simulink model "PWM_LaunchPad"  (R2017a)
settings: Solver=FixedStepDiscrete  StartTime=0.0  StopTime=inf  RelTol=1e-3  EnableMultiTasking=on
undefined symbols (not defined in the file): A, Compare, conversion, DCAEVT1, DCAEVT1FILT, Digital, Event, Filtered, GPTRIP1SEL, GPTRIP2SEL, input, Module, of, start, Trip, TZ1, TZ2, version, Zone
libraries: c2802xlib x5, idelinklib_common x1

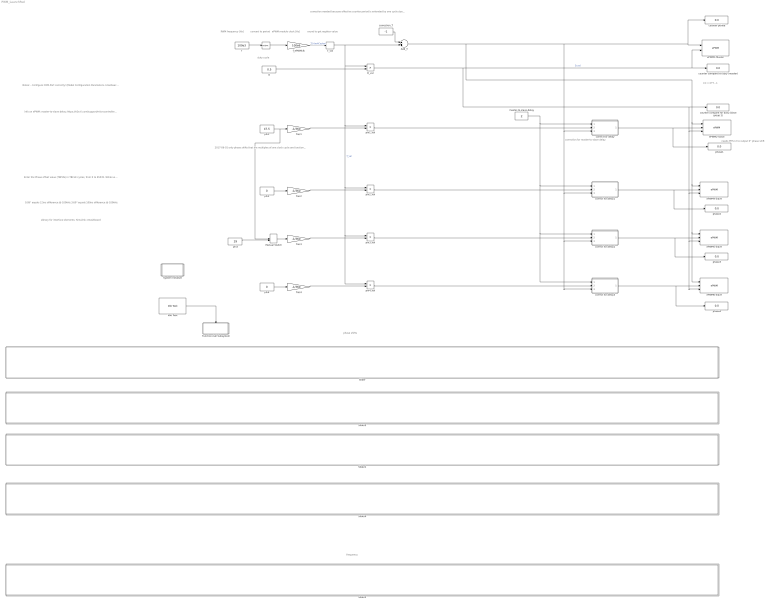
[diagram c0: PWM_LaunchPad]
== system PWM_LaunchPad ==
  note: 2017-06-01 only phase shifts that are multiples of one clock cycle are functioning correctly
  note: correction for master-to-slave delay
  note: needs PHS=2 to output 0° phase shift
  note: info on ePWM: master-to-slave delay: https://e2e.ti.com/support/microcontrollers/c2000/f/171/p/279536/976108 lagging phase-shift: http://e2e.ti.com/support/microcontrollers/c2000/f/171/p/582633/2143131
  note: PWM frequency [Hz]
  note: convert to period
  note: CC = D*T - 1
  note: phase shifts
  note: Library for interface elements: Simulink->Dashboard
  note: Notes: - Configure COM-Port correctly! (Model Configuration Parameters->Hardware Implementation->Groups:External Mode->Serial port) COM-Port Number taken from Windows device manager - In model settings -> Hardware Implementation, disable "Boot from flash" (unnecessary, only slows down program download)
  note: 0.09° equals 2.5ns difference @ 100kHz 3.60° equals 100ns difference @ 100kHz
  note: Enter the Phase offset value (TBPHS) in TBCLK cycles, from 0 to 65535. While using HRPWM, you may enter decimal values The Extension Register for the HRPWM Period (TBPRDHR) provides an 8 bit representation of the decimal part
  note: frequency
  note: correction needed because effective counter period is extended by one cycle due to counter reload See ePWM RefGuide, p. 89, Example 14
  note: ePWM module clock [Hz]
  note: round to get register value
  note: duty cycle
  Add_T : Sum
  D : Constant  Value=0.5
  D_val : Product
  Function-Call Subsystem : Subsystem  TreatAsAtomicUnit=on
  Idle Task : idelinklib_common/Idle Task  tasknumbers=[1]  taskpriorities=100017  taskpreempts=[0]  showinput=off  simPriority=0
  Manual Switch : ManualSwitch
  Slider : Subsystem  DialogController=hmiCreateDDGDialog  IsWebBlock=on
  Slider1 : Subsystem  DialogController=hmiCreateDDGDialog  IsWebBlock=on
  Slider2 : Subsystem  DialogController=hmiCreateDDGDialog  IsWebBlock=on
  Slider3 : Subsystem  DialogController=hmiCreateDDGDialog  IsWebBlock=on
  Slider4 : Subsystem  DialogController=hmiCreateDDGDialog  IsWebBlock=on
  System Initialize : Subsystem
  T : Math  Operator=reciprocal
  T_val : Rounding
  correct for delay : Subsystem
  correct for delay1 : Subsystem
  correct for delay2 : Subsystem
  correct for delay3 : Subsystem
  correction_T : Constant  Value=-1
  counter compare for duty (master) : Display
  counter compare for duty (slave group 1) : Display
  counter period : Display
  ePWM1-Master : c2802xlib/ePWM  useModule=ePWM1  ePWMxLINKTBPRD=Not Linked  periodUnits=Clock cycles  timerSource=Input port  timerPeriod_clk=0  timerPeriod_sec=10e-3  tbshadow=Counter equals to zero  countingMode=Up  phaseActiveEnable=Disable  phaseDirection=Count down after sync  phaseActive=0  synchronizationEnable=off  dcaevt1Sync=off  dcbevt1Sync=off  synchronizationOption=Counter equals to zero (CTR=Zero)  clockPrescale=1  HSclockPrescale=1  enswap=off  ePWMxAStatus=on  ePWMxAactionLogic1=Set  ePWMxAactionLogic2=Do nothing  ePWMxAactionLogic3=Clear  ePWMxAactionLogic4=Clear  ePWMxAactionLogic5=Do nothing  ePWMxAactionLogic6=Do nothing  ePWMxALoadMode=Load on counter equals to zero (CTR=Zero)  ePWMxACSFenable=off  ePWMxACSFvalue=Forcing disable  ePWMxASFreload=Zero  ePWMxBStatus=off  ePWMxBactionLogic1=Do nothing  ePWMxBactionLogic2=Do nothing  ePWMxBactionLogic3=Do nothing  ePWMxBactionLogic4=Do nothing  ePWMxBactionLogic5=Do nothing  ePWMxBactionLogic6=Do nothing  ePWMxBLoadMode=Load on counter equals to zero (CTR=Zero)  ePWMxBCSFenable=off  ePWMxBCSFvalue=Forcing disable  ePWMxBSFreload=Zero  ePWNxBOutWay=off  ePWMxLINKCMPA=Not Linked  CMPAUnits=Clock cycles  CMPASource=Input port  CMPAValue_per=50  CMPAValue_clk=0  enCMPAshadow=Counter equals to zero  ePWMxLINKCMPB=Not Linked  CMPBUnits=Clock cycles  CMPBSource=Specify via dialog  CMPBValue_per=50  CMPBValue_clk=0  enCMPBshadow=Counter equals to zero  ePWMxLINKCMPC=Not Linked  CMPCUnits=Clock cycles  CMPCSource=Specify via dialog  CMPCValue_per=50  CMPCValue_clk=0  enCMPCshadow=Counter equals to zero  ePWMxLINKCMPD=Not Linked  CMPDUnits=Clock cycles  CMPDSource=Specify via dialog  CMPDValue_per=50  CMPDValue_clk=0  enCMPDshadow=Counter equals to zero  enableDBePWMxA=off  enableDBePWMxB=off  enhalfcycle=off  DBpolarity=Active high (AH)  DBedgeDelay=Positive  DBSource_ePWMxA=ePWMxA  DBSource_ePWMxB=ePWMxA  DBperiodSource=Specify via dialog  REDperiod=0  FEDperiod=0  adcstartModuleA=off  adcrequestEventA=First event  adcstartEventA=Digital Compare Module A Event 1 start of conversion (DCAEVT1.soc)  adcstartEventA_type2=Counter equals to period (CTR=PRD)  adcstartModuleB=off  adcrequestEventB=First event  adcstartEventB=Counter equals to zero (CTR=Zero)  adcstartEventB_type2=Counter equals to zero (CTR=Zero)  intEn=off  intPrd=First event  intSel=Counter equals to zero (CTR=Zero)  intSel_type2=Counter equals to zero (CTR=Zero)  hrpe=off  enHRPWM=on  HRPWM_LoadMode=Counter equals to zero (CTR=ZERO)  HRPWM_CTLMode=Phase control mode  HRPWM_EDGMode=Both edge  hrpeb=off  enHRPWMB=off  HRPWM_LoadModeB=Counter equals to zero (CTR=ZERO)  HRPWM_CTLModeB=Duty or Period control mode  HRPWM_EDGModeB=Both edge  enSFO=on  enautoconv=on  chopperEnable=off  chopperFrequency=1  chopperFirstwidth=1  chopperDuty=12.5%  tripZonesource=Specify via dialog  tzselOSHT1=off  tzselOSHT2=off  tzselOSHT3=off  tzselOSHDCAEV1=off  tzselOSHDCBEV1=off  tzselCBC1=off  tzselCBC2=off  tzselCBC3=off  tzselCBCDCAEV2=off  tzselCBCDCBEV2=off  tzselOSHT4=off  tzselOSHT5=off  tzselOSHT6=off  tzselCBC4=off  tzselCBC5=off  tzselCBC6=off  enTzOstIntr=off  enTzCbcIntr=off  enTzDCAEVT1Intr=off  enTzDCAEVT2Intr=off  enTzDCBEVT1Intr=off  enTzDCBEVT2Intr=off  ePWMxAforced=No action  ePWMxBforced=No action  DCAEVT1forced=No action  DCBEVT1forced=No action  DCAEVT2forced=No action  DCBEVT2forced=No action  dcah=Trip Zone 1 input (TZ1)  dcal=Trip Zone 2 input (TZ2)  dcbh=Trip Zone 1 input (TZ1)  dcbl=Trip Zone 2 input (TZ2)  dcah_type2=GPTRIP1SEL/(TZ1)  dcal_type2=GPTRIP2SEL/(TZ2)  dcbh_type2=GPTRIP1SEL/(TZ1)  dcbl_type2=GPTRIP2SEL/(TZ2)  gendcaevt1=Event disabled  gendcaevt2=Event disabled  gendcbevt1=Event disabled  gendcbevt2=Event disabled  dcaevt1src=DCAEVT1 with sync  dcaevt2src=DCAEVT2 with sync  dcbevt1src=DCBEVT1 with sync  dcbevt2src=DCBEVT2 with sync  pulsesel=Counter equals to zero (CTR=Zero)  blankinv=off  blankoffset=0  blankwidth=0  evsrcsel=Filtered version of DCAEVT1 (DCAEVT1FILT)  encape=off  PwmType=C2000_Type4
  ePWM2-Slave : c2802xlib/ePWM  useModule=ePWM2  ePWMxLINKTBPRD=Not Linked  periodUnits=Clock cycles  timerSource=Input port  timerPeriod_clk=500  timerPeriod_sec=10e-3  tbshadow=Counter equals to zero  countingMode=Up  phaseActiveEnable=Set counter to phase value specified via input port  phaseDirection=Count down after sync  phaseActive=0  synchronizationEnable=off  dcaevt1Sync=off  dcbevt1Sync=off  synchronizationOption=Pass through (EPWMxSYNCI or SWFSYNC)  clockPrescale=1  HSclockPrescale=1  enswap=off  ePWMxAStatus=on  ePWMxAactionLogic1=Set  ePWMxAactionLogic2=Do nothing  ePWMxAactionLogic3=Clear  ePWMxAactionLogic4=Clear  ePWMxAactionLogic5=Do nothing  ePWMxAactionLogic6=Do nothing  ePWMxALoadMode=Load on counter equals to zero (CTR=Zero)  ePWMxACSFenable=off  ePWMxACSFvalue=Forcing disable  ePWMxASFreload=Zero  ePWMxBStatus=off  ePWMxBactionLogic1=Do nothing  ePWMxBactionLogic2=Do nothing  ePWMxBactionLogic3=Do nothing  ePWMxBactionLogic4=Do nothing  ePWMxBactionLogic5=Do nothing  ePWMxBactionLogic6=Do nothing  ePWMxBLoadMode=Load on counter equals to zero (CTR=Zero)  ePWMxBCSFenable=off  ePWMxBCSFvalue=Forcing disable  ePWMxBSFreload=Zero  ePWNxBOutWay=off  ePWMxLINKCMPA=Not Linked  CMPAUnits=Clock cycles  CMPASource=Input port  CMPAValue_per=50  CMPAValue_clk=500  enCMPAshadow=Counter equals to zero  ePWMxLINKCMPB=Not Linked  CMPBUnits=Clock cycles  CMPBSource=Specify via dialog  CMPBValue_per=50  CMPBValue_clk=0  enCMPBshadow=Counter equals to zero  ePWMxLINKCMPC=Not Linked  CMPCUnits=Clock cycles  CMPCSource=Specify via dialog  CMPCValue_per=50  CMPCValue_clk=0  enCMPCshadow=Counter equals to zero  ePWMxLINKCMPD=Not Linked  CMPDUnits=Clock cycles  CMPDSource=Specify via dialog  CMPDValue_per=50  CMPDValue_clk=0  enCMPDshadow=Counter equals to zero  enableDBePWMxA=off  enableDBePWMxB=off  enhalfcycle=off  DBpolarity=Active high (AH)  DBedgeDelay=Positive  DBSource_ePWMxA=ePWMxA  DBSource_ePWMxB=ePWMxA  DBperiodSource=Specify via dialog  REDperiod=0  FEDperiod=0  adcstartModuleA=off  adcrequestEventA=First event  adcstartEventA=Digital Compare Module A Event 1 start of conversion (DCAEVT1.soc)  adcstartEventA_type2=Counter equals to period (CTR=PRD)  adcstartModuleB=off  adcrequestEventB=First event  adcstartEventB=Counter equals to zero (CTR=Zero)  adcstartEventB_type2=Counter equals to zero (CTR=Zero)  intEn=off  intPrd=First event  intSel=Counter equals to zero (CTR=Zero)  intSel_type2=Counter equals to zero (CTR=Zero)  hrpe=off  enHRPWM=on  HRPWM_LoadMode=Counter equals to zero (CTR=ZERO)  HRPWM_CTLMode=Phase control mode  HRPWM_EDGMode=Both edge  hrpeb=off  enHRPWMB=off  HRPWM_LoadModeB=Counter equals to zero (CTR=ZERO)  HRPWM_CTLModeB=Duty or Period control mode  HRPWM_EDGModeB=Both edge  enSFO=on  enautoconv=on  chopperEnable=off  chopperFrequency=1  chopperFirstwidth=1  chopperDuty=12.5%  tripZonesource=Specify via dialog  tzselOSHT1=off  tzselOSHT2=off  tzselOSHT3=off  tzselOSHDCAEV1=off  tzselOSHDCBEV1=off  tzselCBC1=off  tzselCBC2=off  tzselCBC3=off  tzselCBCDCAEV2=off  tzselCBCDCBEV2=off  tzselOSHT4=off  tzselOSHT5=off  tzselOSHT6=off  tzselCBC4=off  tzselCBC5=off  tzselCBC6=off  enTzOstIntr=off  enTzCbcIntr=off  enTzDCAEVT1Intr=off  enTzDCAEVT2Intr=off  enTzDCBEVT1Intr=off  enTzDCBEVT2Intr=off  ePWMxAforced=No action  ePWMxBforced=No action  DCAEVT1forced=No action  DCBEVT1forced=No action  DCAEVT2forced=No action  DCBEVT2forced=No action  dcah=Trip Zone 1 input (TZ1)  dcal=Trip Zone 2 input (TZ2)  dcbh=Trip Zone 1 input (TZ1)  dcbl=Trip Zone 2 input (TZ2)  dcah_type2=GPTRIP1SEL/(TZ1)  dcal_type2=GPTRIP2SEL/(TZ2)  dcbh_type2=GPTRIP1SEL/(TZ1)  dcbl_type2=GPTRIP2SEL/(TZ2)  gendcaevt1=Event disabled  gendcaevt2=Event disabled  gendcbevt1=Event disabled  gendcbevt2=Event disabled  dcaevt1src=DCAEVT1 with sync  dcaevt2src=DCAEVT2 with sync  dcbevt1src=DCBEVT1 with sync  dcbevt2src=DCBEVT2 with sync  pulsesel=Counter equals to zero (CTR=Zero)  blankinv=off  blankoffset=0  blankwidth=0  evsrcsel=Filtered version of DCAEVT1 (DCAEVT1FILT)  encape=off  PwmType=C2000_Type4
  ePWM4-Slave : c2802xlib/ePWM  useModule=ePWM4  ePWMxLINKTBPRD=Not Linked  periodUnits=Clock cycles  timerSource=Input port  timerPeriod_clk=500  timerPeriod_sec=10e-3  tbshadow=Counter equals to zero  countingMode=Up  phaseActiveEnable=Set counter to phase value specified via input port  phaseDirection=Count down after sync  phaseActive=0  synchronizationEnable=off  dcaevt1Sync=off  dcbevt1Sync=off  synchronizationOption=Pass through (EPWMxSYNCI or SWFSYNC)  clockPrescale=1  HSclockPrescale=1  enswap=off  ePWMxAStatus=on  ePWMxAactionLogic1=Set  ePWMxAactionLogic2=Do nothing  ePWMxAactionLogic3=Clear  ePWMxAactionLogic4=Clear  ePWMxAactionLogic5=Do nothing  ePWMxAactionLogic6=Do nothing  ePWMxALoadMode=Load on counter equals to zero (CTR=Zero)  ePWMxACSFenable=off  ePWMxACSFvalue=Forcing disable  ePWMxASFreload=Zero  ePWMxBStatus=off  ePWMxBactionLogic1=Do nothing  ePWMxBactionLogic2=Do nothing  ePWMxBactionLogic3=Do nothing  ePWMxBactionLogic4=Do nothing  ePWMxBactionLogic5=Do nothing  ePWMxBactionLogic6=Do nothing  ePWMxBLoadMode=Load on counter equals to zero (CTR=Zero)  ePWMxBCSFenable=off  ePWMxBCSFvalue=Forcing disable  ePWMxBSFreload=Zero  ePWNxBOutWay=off  ePWMxLINKCMPA=Not Linked  CMPAUnits=Clock cycles  CMPASource=Input port  CMPAValue_per=50  CMPAValue_clk=500  enCMPAshadow=Counter equals to zero  ePWMxLINKCMPB=Not Linked  CMPBUnits=Clock cycles  CMPBSource=Specify via dialog  CMPBValue_per=50  CMPBValue_clk=0  enCMPBshadow=Counter equals to zero  ePWMxLINKCMPC=Not Linked  CMPCUnits=Clock cycles  CMPCSource=Specify via dialog  CMPCValue_per=50  CMPCValue_clk=0  enCMPCshadow=Counter equals to zero  ePWMxLINKCMPD=Not Linked  CMPDUnits=Clock cycles  CMPDSource=Specify via dialog  CMPDValue_per=50  CMPDValue_clk=0  enCMPDshadow=Counter equals to zero  enableDBePWMxA=off  enableDBePWMxB=off  enhalfcycle=off  DBpolarity=Active high (AH)  DBedgeDelay=Positive  DBSource_ePWMxA=ePWMxA  DBSource_ePWMxB=ePWMxA  DBperiodSource=Specify via dialog  REDperiod=0  FEDperiod=0  adcstartModuleA=off  adcrequestEventA=First event  adcstartEventA=Digital Compare Module A Event 1 start of conversion (DCAEVT1.soc)  adcstartEventA_type2=Counter equals to period (CTR=PRD)  adcstartModuleB=off  adcrequestEventB=First event  adcstartEventB=Counter equals to zero (CTR=Zero)  adcstartEventB_type2=Counter equals to zero (CTR=Zero)  intEn=off  intPrd=First event  intSel=Counter equals to zero (CTR=Zero)  intSel_type2=Counter equals to zero (CTR=Zero)  hrpe=off  enHRPWM=on  HRPWM_LoadMode=Counter equals to zero (CTR=ZERO)  HRPWM_CTLMode=Phase control mode  HRPWM_EDGMode=Both edge  hrpeb=off  enHRPWMB=off  HRPWM_LoadModeB=Counter equals to zero (CTR=ZERO)  HRPWM_CTLModeB=Duty or Period control mode  HRPWM_EDGModeB=Both edge  enSFO=on  enautoconv=on  chopperEnable=off  chopperFrequency=1  chopperFirstwidth=1  chopperDuty=12.5%  tripZonesource=Specify via dialog  tzselOSHT1=off  tzselOSHT2=off  tzselOSHT3=off  tzselOSHDCAEV1=off  tzselOSHDCBEV1=off  tzselCBC1=off  tzselCBC2=off  tzselCBC3=off  tzselCBCDCAEV2=off  tzselCBCDCBEV2=off  tzselOSHT4=off  tzselOSHT5=off  tzselOSHT6=off  tzselCBC4=off  tzselCBC5=off  tzselCBC6=off  enTzOstIntr=off  enTzCbcIntr=off  enTzDCAEVT1Intr=off  enTzDCAEVT2Intr=off  enTzDCBEVT1Intr=off  enTzDCBEVT2Intr=off  ePWMxAforced=No action  ePWMxBforced=No action  DCAEVT1forced=No action  DCBEVT1forced=No action  DCAEVT2forced=No action  DCBEVT2forced=No action  dcah=Trip Zone 1 input (TZ1)  dcal=Trip Zone 2 input (TZ2)  dcbh=Trip Zone 1 input (TZ1)  dcbl=Trip Zone 2 input (TZ2)  dcah_type2=GPTRIP1SEL/(TZ1)  dcal_type2=GPTRIP2SEL/(TZ2)  dcbh_type2=GPTRIP1SEL/(TZ1)  dcbl_type2=GPTRIP2SEL/(TZ2)  gendcaevt1=Event disabled  gendcaevt2=Event disabled  gendcbevt1=Event disabled  gendcbevt2=Event disabled  dcaevt1src=DCAEVT1 with sync  dcaevt2src=DCAEVT2 with sync  dcbevt1src=DCBEVT1 with sync  dcbevt2src=DCBEVT2 with sync  pulsesel=Counter equals to zero (CTR=Zero)  blankinv=off  blankoffset=0  blankwidth=0  evsrcsel=Filtered version of DCAEVT1 (DCAEVT1FILT)  encape=off  PwmType=C2000_Type4
  ePWM5-Slave : c2802xlib/ePWM  useModule=ePWM5  ePWMxLINKTBPRD=Not Linked  periodUnits=Clock cycles  timerSource=Input port  timerPeriod_clk=500  timerPeriod_sec=10e-3  tbshadow=Counter equals to zero  countingMode=Up  phaseActiveEnable=Set counter to phase value specified via input port  phaseDirection=Count down after sync  phaseActive=10.25  synchronizationEnable=off  dcaevt1Sync=off  dcbevt1Sync=off  synchronizationOption=Pass through (EPWMxSYNCI or SWFSYNC)  clockPrescale=1  HSclockPrescale=1  enswap=off  ePWMxAStatus=on  ePWMxAactionLogic1=Set  ePWMxAactionLogic2=Do nothing  ePWMxAactionLogic3=Clear  ePWMxAactionLogic4=Clear  ePWMxAactionLogic5=Do nothing  ePWMxAactionLogic6=Do nothing  ePWMxALoadMode=Load on counter equals to zero (CTR=Zero)  ePWMxACSFenable=off  ePWMxACSFvalue=Forcing disable  ePWMxASFreload=Zero  ePWMxBStatus=off  ePWMxBactionLogic1=Do nothing  ePWMxBactionLogic2=Do nothing  ePWMxBactionLogic3=Do nothing  ePWMxBactionLogic4=Do nothing  ePWMxBactionLogic5=Do nothing  ePWMxBactionLogic6=Do nothing  ePWMxBLoadMode=Load on counter equals to zero (CTR=Zero)  ePWMxBCSFenable=off  ePWMxBCSFvalue=Forcing disable  ePWMxBSFreload=Zero  ePWNxBOutWay=off  ePWMxLINKCMPA=Not Linked  CMPAUnits=Clock cycles  CMPASource=Input port  CMPAValue_per=50  CMPAValue_clk=500  enCMPAshadow=Counter equals to zero  ePWMxLINKCMPB=Not Linked  CMPBUnits=Clock cycles  CMPBSource=Specify via dialog  CMPBValue_per=50  CMPBValue_clk=0  enCMPBshadow=Counter equals to zero  ePWMxLINKCMPC=Not Linked  CMPCUnits=Clock cycles  CMPCSource=Specify via dialog  CMPCValue_per=50  CMPCValue_clk=0  enCMPCshadow=Counter equals to zero  ePWMxLINKCMPD=Not Linked  CMPDUnits=Clock cycles  CMPDSource=Specify via dialog  CMPDValue_per=50  CMPDValue_clk=0  enCMPDshadow=Counter equals to zero  enableDBePWMxA=off  enableDBePWMxB=off  enhalfcycle=off  DBpolarity=Active high (AH)  DBedgeDelay=Positive  DBSource_ePWMxA=ePWMxA  DBSource_ePWMxB=ePWMxA  DBperiodSource=Specify via dialog  REDperiod=0  FEDperiod=0  adcstartModuleA=off  adcrequestEventA=First event  adcstartEventA=Digital Compare Module A Event 1 start of conversion (DCAEVT1.soc)  adcstartEventA_type2=Counter equals to period (CTR=PRD)  adcstartModuleB=off  adcrequestEventB=First event  adcstartEventB=Counter equals to zero (CTR=Zero)  adcstartEventB_type2=Counter equals to zero (CTR=Zero)  intEn=off  intPrd=First event  intSel=Counter equals to zero (CTR=Zero)  intSel_type2=Counter equals to zero (CTR=Zero)  hrpe=off  enHRPWM=on  HRPWM_LoadMode=Counter equals to zero (CTR=ZERO)  HRPWM_CTLMode=Phase control mode  HRPWM_EDGMode=Both edge  hrpeb=off  enHRPWMB=off  HRPWM_LoadModeB=Counter equals to zero (CTR=ZERO)  HRPWM_CTLModeB=Duty or Period control mode  HRPWM_EDGModeB=Both edge  enSFO=on  enautoconv=on  chopperEnable=off  chopperFrequency=1  chopperFirstwidth=1  chopperDuty=12.5%  tripZonesource=Specify via dialog  tzselOSHT1=off  tzselOSHT2=off  tzselOSHT3=off  tzselOSHDCAEV1=off  tzselOSHDCBEV1=off  tzselCBC1=off  tzselCBC2=off  tzselCBC3=off  tzselCBCDCAEV2=off  tzselCBCDCBEV2=off  tzselOSHT4=off  tzselOSHT5=off  tzselOSHT6=off  tzselCBC4=off  tzselCBC5=off  tzselCBC6=off  enTzOstIntr=off  enTzCbcIntr=off  enTzDCAEVT1Intr=off  enTzDCAEVT2Intr=off  enTzDCBEVT1Intr=off  enTzDCBEVT2Intr=off  ePWMxAforced=No action  ePWMxBforced=No action  DCAEVT1forced=No action  DCBEVT1forced=No action  DCAEVT2forced=No action  DCBEVT2forced=No action  dcah=Trip Zone 1 input (TZ1)  dcal=Trip Zone 2 input (TZ2)  dcbh=Trip Zone 1 input (TZ1)  dcbl=Trip Zone 2 input (TZ2)  dcah_type2=GPTRIP1SEL/(TZ1)  dcal_type2=GPTRIP2SEL/(TZ2)  dcbh_type2=GPTRIP1SEL/(TZ1)  dcbl_type2=GPTRIP2SEL/(TZ2)  gendcaevt1=Event disabled  gendcaevt2=Event disabled  gendcbevt1=Event disabled  gendcbevt2=Event disabled  dcaevt1src=DCAEVT1 with sync  dcaevt2src=DCAEVT2 with sync  dcbevt1src=DCBEVT1 with sync  dcbevt2src=DCBEVT2 with sync  pulsesel=Counter equals to zero (CTR=Zero)  blankinv=off  blankoffset=0  blankwidth=0  evsrcsel=Filtered version of DCAEVT1 (DCAEVT1FILT)  encape=off  PwmType=C2000_Type4
  ePWM6-Slave : c2802xlib/ePWM  useModule=ePWM6  ePWMxLINKTBPRD=Not Linked  periodUnits=Clock cycles  timerSource=Input port  timerPeriod_clk=500  timerPeriod_sec=10e-3  tbshadow=Counter equals to zero  countingMode=Up  phaseActiveEnable=Set counter to phase value specified via input port  phaseDirection=Count down after sync  phaseActive=10.25  synchronizationEnable=off  dcaevt1Sync=off  dcbevt1Sync=off  synchronizationOption=Pass through (EPWMxSYNCI or SWFSYNC)  clockPrescale=1  HSclockPrescale=1  enswap=off  ePWMxAStatus=on  ePWMxAactionLogic1=Set  ePWMxAactionLogic2=Do nothing  ePWMxAactionLogic3=Clear  ePWMxAactionLogic4=Clear  ePWMxAactionLogic5=Do nothing  ePWMxAactionLogic6=Do nothing  ePWMxALoadMode=Load on counter equals to zero (CTR=Zero)  ePWMxACSFenable=off  ePWMxACSFvalue=Forcing disable  ePWMxASFreload=Zero  ePWMxBStatus=off  ePWMxBactionLogic1=Do nothing  ePWMxBactionLogic2=Do nothing  ePWMxBactionLogic3=Do nothing  ePWMxBactionLogic4=Do nothing  ePWMxBactionLogic5=Do nothing  ePWMxBactionLogic6=Do nothing  ePWMxBLoadMode=Load on counter equals to zero (CTR=Zero)  ePWMxBCSFenable=off  ePWMxBCSFvalue=Forcing disable  ePWMxBSFreload=Zero  ePWNxBOutWay=off  ePWMxLINKCMPA=Not Linked  CMPAUnits=Clock cycles  CMPASource=Input port  CMPAValue_per=50  CMPAValue_clk=500  enCMPAshadow=Counter equals to zero  ePWMxLINKCMPB=Not Linked  CMPBUnits=Clock cycles  CMPBSource=Specify via dialog  CMPBValue_per=50  CMPBValue_clk=0  enCMPBshadow=Counter equals to zero  ePWMxLINKCMPC=Not Linked  CMPCUnits=Clock cycles  CMPCSource=Specify via dialog  CMPCValue_per=50  CMPCValue_clk=0  enCMPCshadow=Counter equals to zero  ePWMxLINKCMPD=Not Linked  CMPDUnits=Clock cycles  CMPDSource=Specify via dialog  CMPDValue_per=50  CMPDValue_clk=0  enCMPDshadow=Counter equals to zero  enableDBePWMxA=off  enableDBePWMxB=off  enhalfcycle=off  DBpolarity=Active high (AH)  DBedgeDelay=Positive  DBSource_ePWMxA=ePWMxA  DBSource_ePWMxB=ePWMxA  DBperiodSource=Specify via dialog  REDperiod=0  FEDperiod=0  adcstartModuleA=off  adcrequestEventA=First event  adcstartEventA=Digital Compare Module A Event 1 start of conversion (DCAEVT1.soc)  adcstartEventA_type2=Counter equals to period (CTR=PRD)  adcstartModuleB=off  adcrequestEventB=First event  adcstartEventB=Counter equals to zero (CTR=Zero)  adcstartEventB_type2=Counter equals to zero (CTR=Zero)  intEn=off  intPrd=First event  intSel=Counter equals to zero (CTR=Zero)  intSel_type2=Counter equals to zero (CTR=Zero)  hrpe=off  enHRPWM=on  HRPWM_LoadMode=Counter equals to zero (CTR=ZERO)  HRPWM_CTLMode=Phase control mode  HRPWM_EDGMode=Both edge  hrpeb=off  enHRPWMB=off  HRPWM_LoadModeB=Counter equals to zero (CTR=ZERO)  HRPWM_CTLModeB=Duty or Period control mode  HRPWM_EDGModeB=Both edge  enSFO=on  enautoconv=on  chopperEnable=off  chopperFrequency=1  chopperFirstwidth=1  chopperDuty=12.5%  tripZonesource=Specify via dialog  tzselOSHT1=off  tzselOSHT2=off  tzselOSHT3=off  tzselOSHDCAEV1=off  tzselOSHDCBEV1=off  tzselCBC1=off  tzselCBC2=off  tzselCBC3=off  tzselCBCDCAEV2=off  tzselCBCDCBEV2=off  tzselOSHT4=off  tzselOSHT5=off  tzselOSHT6=off  tzselCBC4=off  tzselCBC5=off  tzselCBC6=off  enTzOstIntr=off  enTzCbcIntr=off  enTzDCAEVT1Intr=off  enTzDCAEVT2Intr=off  enTzDCBEVT1Intr=off  enTzDCBEVT2Intr=off  ePWMxAforced=No action  ePWMxBforced=No action  DCAEVT1forced=No action  DCBEVT1forced=No action  DCAEVT2forced=No action  DCBEVT2forced=No action  dcah=Trip Zone 1 input (TZ1)  dcal=Trip Zone 2 input (TZ2)  dcbh=Trip Zone 1 input (TZ1)  dcbl=Trip Zone 2 input (TZ2)  dcah_type2=GPTRIP1SEL/(TZ1)  dcal_type2=GPTRIP2SEL/(TZ2)  dcbh_type2=GPTRIP1SEL/(TZ1)  dcbl_type2=GPTRIP2SEL/(TZ2)  gendcaevt1=Event disabled  gendcaevt2=Event disabled  gendcbevt1=Event disabled  gendcbevt2=Event disabled  dcaevt1src=DCAEVT1 with sync  dcaevt2src=DCAEVT2 with sync  dcbevt1src=DCBEVT1 with sync  dcbevt2src=DCBEVT2 with sync  pulsesel=Counter equals to zero (CTR=Zero)  blankinv=off  blankoffset=0  blankwidth=0  evsrcsel=Filtered version of DCAEVT1 (DCAEVT1FILT)  encape=off  PwmType=C2000_Type4
  f : Constant  Value=100e3
  f_ePWMclk : Gain  Gain=100e6
  frac{1..4} (4 alike) : Gain  Gain=-1/360
  master-to-slave-delay : Constant  Value=2
  phase{1..4} (4 alike) : Display
  phi1 : Constant  Value=47.5
  phi1_val : Product
  phi2 : Constant  Value=0
  phi2_val : Product
  phi3 : Constant  Value=29
  phi3_val : Product
  phi4 : Constant  Value=0
  phi4_val : Product
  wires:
  T/1 -> f_ePWMclk/1
  phi2/1 -> frac2/1
  frac2/1 -> phi2_val/2
  f_ePWMclk/1 -> T_val/1  "T [clockCycles]"
  frac3/1 -> phi3_val/2
  correction_T/1 -> Add_T/1
  D_val/1 -> ePWM1-Master/2, counter compare for duty (master)/1, ePWM6-Slave/3, ePWM5-Slave/3, ePWM4-Slave/3, ePWM2-Slave/3, counter compare for duty (slave group 1)/1  "D_val"
  phi4/1 -> frac4/1
  frac4/1 -> phi4_val/2
  T_val/1 -> D_val/1, phi4_val/1, phi3_val/1, phi2_val/1, phi1_val/1, Add_T/2  "T_val"
  f/1 -> T/1
  D/1 -> D_val/2
  phi1/1 -> Manual Switch/1, frac1/1
  frac1/1 -> phi1_val/2
  Add_T/1 -> ePWM6-Slave/1, ePWM5-Slave/1, ePWM4-Slave/1, ePWM2-Slave/1, correct for delay3/3(max), correct for delay2/3(max), correct for delay1/3(max), correct for delay/3(max), ePWM1-Master/1, counter period/1
  master-to-slave-delay/1 -> correct for delay1/1(delay), correct for delay3/1(delay), correct for delay2/1(delay), correct for delay/1(delay)
  Idle Task/1 -> Function-Call Subsystem/Trigger
  correct for delay/1(correct val) -> phase1/1, ePWM2-Slave/2
  correct for delay1/1(correct val) -> phase2/1, ePWM4-Slave/2
  correct for delay2/1(correct val) -> phase3/1, ePWM5-Slave/2
  correct for delay3/1(correct val) -> phase4/1, ePWM6-Slave/2
  phi1_val/1 -> correct for delay/2(shift)
  phi2_val/1 -> correct for delay1/2(shift)
  phi3_val/1 -> correct for delay2/2(shift)
  phi4_val/1 -> correct for delay3/2(shift)
  Manual Switch/1 -> frac3/1
  phi3/1 -> Manual Switch/2

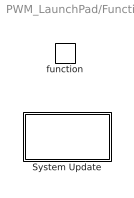
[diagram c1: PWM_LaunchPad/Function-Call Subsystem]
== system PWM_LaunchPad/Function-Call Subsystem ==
  function : TriggerPort  TriggerType=function-call  VariantControl=Variant
  System Update : Subsystem

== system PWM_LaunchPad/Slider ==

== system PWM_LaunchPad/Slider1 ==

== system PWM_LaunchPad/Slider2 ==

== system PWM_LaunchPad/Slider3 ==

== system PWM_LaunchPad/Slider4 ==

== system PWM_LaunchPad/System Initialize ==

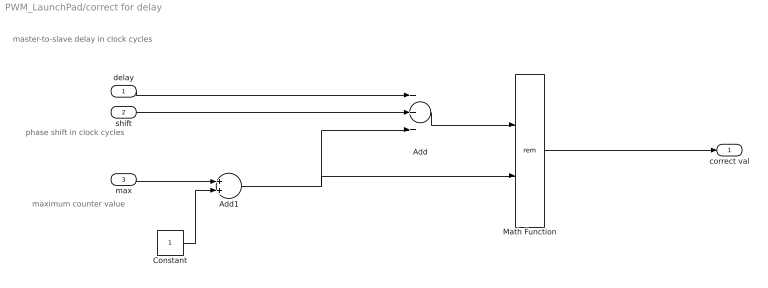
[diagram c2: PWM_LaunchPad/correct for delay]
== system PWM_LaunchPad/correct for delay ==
  note: master-to-slave delay in clock cycles
  note: phase shift in clock cycles
  note: maximum counter value
  delay : Inport
  shift : Inport  Port=2
  max : Inport  Port=3
  Add : Sum  Inputs=+++
  Add1 : Sum
  Constant : Constant
  Math Function : Math  Operator=rem
  correct val : Outport
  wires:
  Add/1 -> Math Function/1
  delay/1 -> Add/1
  shift/1 -> Add/2
  Math Function/1 -> correct val/1
  Constant/1 -> Add1/2
  max/1 -> Add1/1
  Add1/1 -> Math Function/2, Add/3

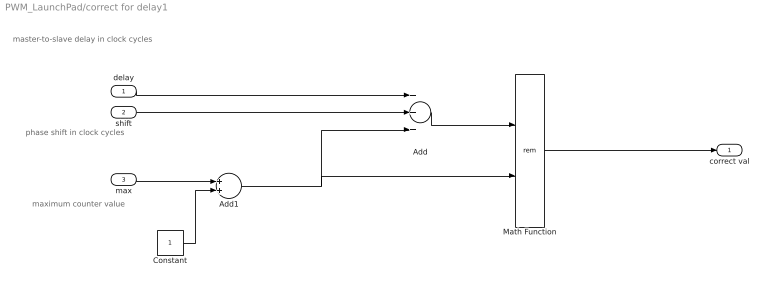
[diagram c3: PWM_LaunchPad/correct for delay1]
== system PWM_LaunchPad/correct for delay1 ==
  note: maximum counter value
  note: phase shift in clock cycles
  note: master-to-slave delay in clock cycles
  delay : Inport
  shift : Inport  Port=2
  max : Inport  Port=3
  Add : Sum  Inputs=+++
  Add1 : Sum
  Constant : Constant
  Math Function : Math  Operator=rem
  correct val : Outport
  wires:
  Add1/1 -> Add/3, Math Function/2
  max/1 -> Add1/1
  Constant/1 -> Add1/2
  Math Function/1 -> correct val/1
  shift/1 -> Add/2
  delay/1 -> Add/1
  Add/1 -> Math Function/1

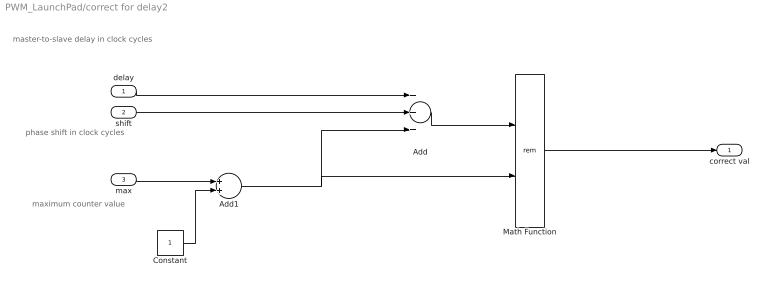
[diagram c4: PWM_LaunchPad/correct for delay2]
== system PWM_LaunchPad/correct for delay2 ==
  note: master-to-slave delay in clock cycles
  note: phase shift in clock cycles
  note: maximum counter value
  delay : Inport
  shift : Inport  Port=2
  max : Inport  Port=3
  Add : Sum  Inputs=+++
  Add1 : Sum
  Constant : Constant
  Math Function : Math  Operator=rem
  correct val : Outport
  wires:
  Add/1 -> Math Function/1
  delay/1 -> Add/1
  shift/1 -> Add/2
  Math Function/1 -> correct val/1
  Constant/1 -> Add1/2
  max/1 -> Add1/1
  Add1/1 -> Math Function/2, Add/3

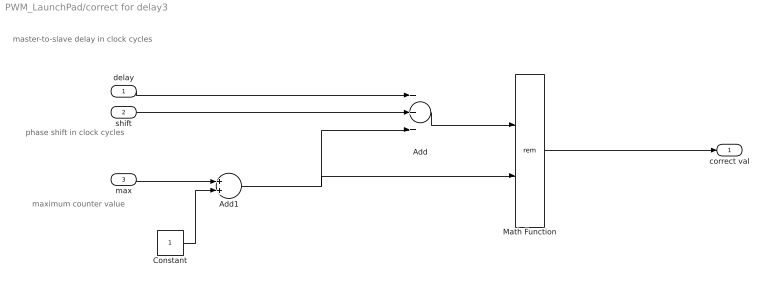
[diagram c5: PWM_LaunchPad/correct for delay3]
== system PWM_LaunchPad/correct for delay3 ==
  note: maximum counter value
  note: phase shift in clock cycles
  note: master-to-slave delay in clock cycles
  delay : Inport
  shift : Inport  Port=2
  max : Inport  Port=3
  Add : Sum  Inputs=+++
  Add1 : Sum
  Constant : Constant
  Math Function : Math  Operator=rem
  correct val : Outport
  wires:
  Add1/1 -> Add/3, Math Function/2
  max/1 -> Add1/1
  Constant/1 -> Add1/2
  Math Function/1 -> correct val/1
  shift/1 -> Add/2
  delay/1 -> Add/1
  Add/1 -> Math Function/1

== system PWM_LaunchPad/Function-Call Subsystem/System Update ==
